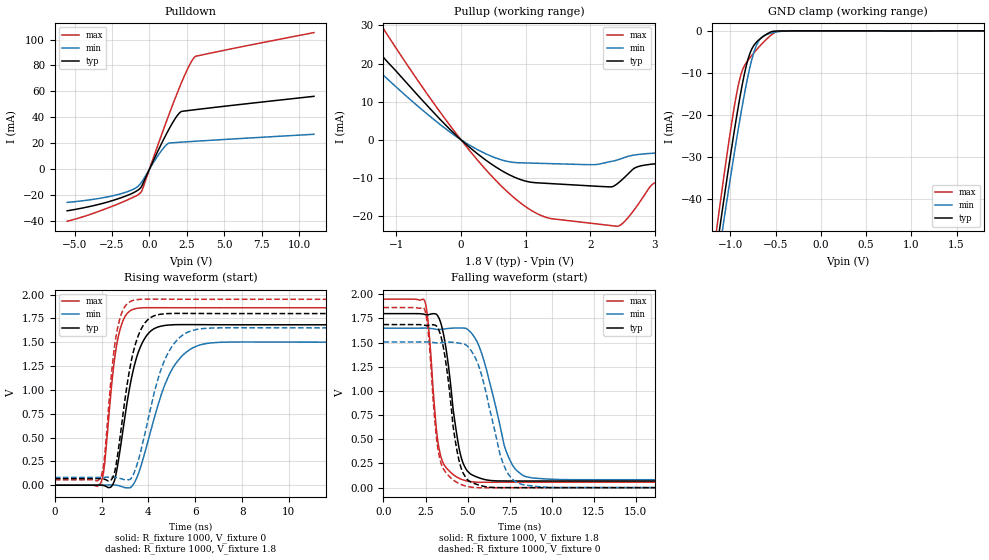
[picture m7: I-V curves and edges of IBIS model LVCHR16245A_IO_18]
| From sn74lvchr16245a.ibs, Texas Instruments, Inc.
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[Model]   LVCHR16245A_IO_18
Model_type  I/O
Vinl=0.5775
Vinh=1.2675
Enable   Active-Low
Vref =   0
Rref =   1000
Cref =   30p
Vmeas =   0.9
| variable   typ   min   max
C_comp   5.51pF   4.99pF   6.47pF
| C_pullup   4.22pF   2.67pF   7.01pF
| C_pulldown   6.14pF   3.77pF   8.58pF
| C_tri-state   5.51pF   4.99pF   6.47pF
[Temperature Range]   40   100   -40
| Ambient temperature   25   85   -40
[Voltage range]   1.8   1.65   1.95
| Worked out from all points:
|   slope of the pulldown table from 0 to 0.27 V, typ, clamps not added: 39.9 ohm
|   slope of the pullup table from 0 to 0.27 V, typ, clamps not added: 69.8 ohm
|   GND clamp passes 1 mA (typ) near -0.61 V on its own axis
|   rising waveform, R_fixture 1000, V_fixture 0: 20-80 % time 735ps typ, 1.18ns min, 472ps max; typ from 0 V to 1.68 V
|   falling waveform, R_fixture 1000, V_fixture 1.8: 20-80 % time 782ps typ, 1.33ns min, 545ps max; typ from 1.8 V to 0.069 V
|   rising waveform, R_fixture 1000, V_fixture 1.8: 20-80 % time 675ps typ, 1.03ns min, 450ps max; typ from 0.069 V to 1.8 V
|   falling waveform, R_fixture 1000, V_fixture 0: 20-80 % time 762ps typ, 1.25ns min, 544ps max; typ from 1.69 V to 0 V
[GND Clamp]
| LVCHR16245A_IO_18
|   Voltage   I(typ)   I(min)   I(max)
-5.5V     -767.2mA   -751.2mA   -793.8mA
-1.145V   -51.21mA   -55.85mA   -46.28mA
-1.12V    -47.45mA   -52.21mA   -42.33mA
-1.075V   -40.76mA   -45.72mA   -35.31mA
-955mV    -23.71mA   -29.04mA   -17.98mA
-885mV    -14.78mA   -19.98mA   -10.62mA
-825mV    -8.476mA   -12.94mA   -7.624mA
-780mV    -5.204mA   -8.392mA   -6.303mA
-715mV    -2.796mA   -3.66mA    -4.625mA
-640mV    -1.39mA    -1.368mA   -2.847mA
-465mV    -40.45uA   -180.4uA   -73.51uA
1.8V      10.89pA    55.22nA    -431pA
[Pulldown]
| LVCHR16245A_IO_18
|   Voltage   I(typ)   I(min)   I(max)
-5.5V     -32.05mA   -25.58mA   -40.14mA
-2.075V   -22.69mA   -19.43mA   -26.68mA
-1.04V    -17.95mA   -15.25mA   -21.4mA
-570mV    -14.09mA   -10.64mA   -17.7mA
-465mV    -11.79mA   -8.989mA   -15.49mA
1V        24.15mA    17.15mA    32.54mA
1.3V      30.76mA    20.12mA    41.93mA
1.795V    40.31mA    20.62mA    56.86mA
2.145V    44.56mA    20.89mA    66.82mA
2.69V     45.4mA     21.3mA     80.56mA
3.055V    45.92mA    21.57mA    86.8mA
11V       56.23mA    26.97mA    105.4mA
[Pullup]
| LVCHR16245A_IO_18
|   Voltage   I(typ)   I(min)   I(max)
-5.5V     122.3mA    25.66mA    160.3mA
-4.815V   105.7mA    29.59mA    138.5mA
-2.06V    39.46mA    31.12mA    52.47mA
-1.635V   30.39mA    23.86mA    40.62mA
-1.24V    22.37mA    17.53mA    30.15mA
385mV     -5.338mA   -3.675mA   -7.843mA
925mV     -10.42mA   -6.005mA   -16.59mA
1.395V    -11.46mA   -6.228mA   -20.63mA
2.43V     -11.3mA    -5.195mA   -22.59mA
2.955V    -6.347mA   -3.51mA    -11.72mA
3.3V      -5.935mA   -3.267mA   -9.915mA
11V       -5.774mA   -3.104mA   -10.4mA
[Ramp]
| LVCHR16245A_IO_18
| variable   typ   min   max
dV/dt_r   1.03/7.51E-10   0.92/1.21E-09   1.12/4.80E-10
dV/dt_f   1.04/7.84E-10   0.94/1.43E-09   1.14/5.68E-10
R_load = 1000
[Rising Waveform]
| LVCHR16245A_IO_18
R_fixture =   1000
C_fixture =   0
L_fixture =   0
V_fixture =   0
V_fixture_min = 0
V_fixture_max = 0
|   Time   V(typ)   V(min)   V(max)
0s        247.3pV    5.549nV    8.466nV
1.975ns   972.6uV    683.8uV    28.17mV
2.13ns    -6.28mV    1.893mV    227.5mV
2.425ns   -11.67mV   3.285mV    1.04V
2.685ns   208.7mV    -1.932mV   1.523V
3.455ns   1.306V     52.49mV    1.852V
4.045ns   1.604V     521.1mV    1.862V
4.955ns   1.681V     1.191V     1.861V
6.51ns    1.683V     1.487V     1.861V
40ns      1.682V     1.5V       1.861V
[Falling Waveform]
| LVCHR16245A_IO_18
R_fixture =   1000
C_fixture =   0
L_fixture =   0
V_fixture =   1.8
V_fixture_min = 1.65
V_fixture_max = 1.95
|   Time   V(typ)   V(min)   V(max)
0s        1.8V       1.65V      1.95V
2.45ns    1.792V     1.65V      1.93V
3.27ns    1.764V     1.636V     438.7mV
3.71ns    1.449V     1.644V     210.8mV
4.485ns   416.7mV    1.652V     98.56mV
4.885ns   199.3mV    1.649V     72.6mV
5.85ns    92.15mV    1.383V     55.81mV
7.39ns    69.04mV    335.6mV    56.81mV
8.48ns    68.84mV    113mV      56.98mV
40ns      68.74mV    81.49mV    56.91mV
[Rising Waveform]
| LVCHR16245A_IO_18
R_fixture =   1000
C_fixture =   0
L_fixture =   0
V_fixture =   1.8
V_fixture_min = 1.65
V_fixture_max = 1.95
|   Time   V(typ)   V(min)   V(max)
0s        68.68mV    81.32mV    56.88mV
1.975ns   69.5mV     81.97mV    87.9mV
2.125ns   62.78mV    83.03mV    297.7mV
2.415ns   57.34mV    84.11mV    1.149V
2.66ns    277.6mV    79.74mV    1.618V
3.44ns    1.475V     163.4mV    1.944V
3.93ns    1.725V     628mV      1.951V
4.705ns   1.798V     1.319V     1.951V
6.1ns     1.801V     1.636V     1.95V
40ns      1.8V       1.65V      1.95V
[Falling Waveform]
| LVCHR16245A_IO_18
R_fixture =   1000
C_fixture =   0
L_fixture =   0
V_fixture =   0
V_fixture_min = 0
V_fixture_max = 0
|   Time   V(typ)   V(min)   V(max)
0s        1.687V     1.507V     1.863V
2.445ns   1.68V      1.507V     1.844V
3.235ns   1.65V      1.496V     404.5mV
3.66ns    1.351V     1.504V     168.2mV
4.365ns   389.8mV    1.499V     54.49mV
4.875ns   110.2mV    1.48V      17.52mV
5.735ns   23.95mV    1.221V     -958.6uV
7.15ns    49.22uV    235.5mV    -233.4uV
8.245ns   229.4uV    33.04mV    77.81uV
40ns      62.52uV    161.6uV    21.82uV
